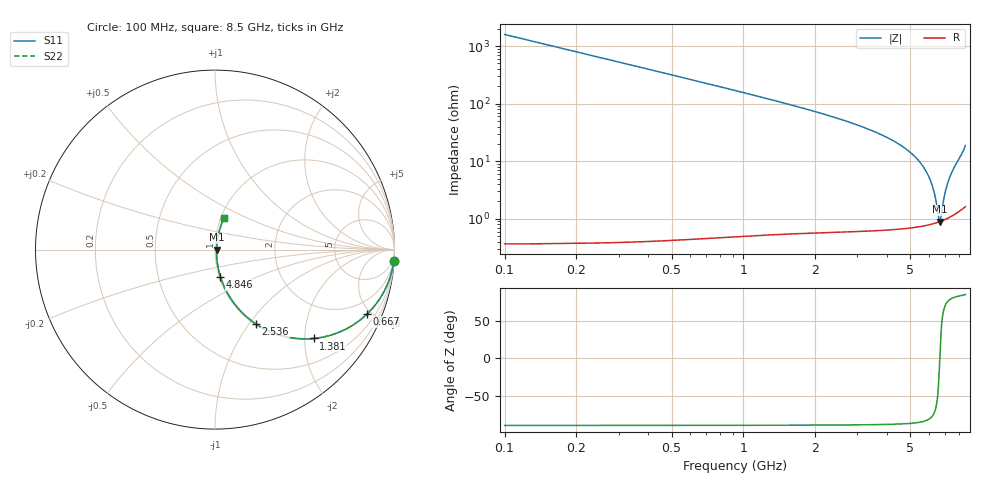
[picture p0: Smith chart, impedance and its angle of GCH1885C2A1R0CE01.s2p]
!Murata Part Number: GCH1885C2A1R0CE01
!These Parameters are Measured in Series Mode Connection
!Data Generated on Jun 19, 2026
!  o--ll--o
!Port1  Port2
!  o------o
!Operation Temp=25[degC], DC Bias Voltage=0[V]
!Freq. Start=100[MHz] Stop=9[GHz] 401[Steps]
# Hz S RI R 50
!Freq.(Hz) S11(Real) S11(Imag) S21(Real) S21(Imag) S12(Real) S12(Imag) S22(Real) S22(Imag)
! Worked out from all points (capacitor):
!   401 points, 100 MHz to 8.5 GHz, reference 50 ohm
!   read as one part in series: C = 1 pF near 142 MHz
!   lowest |Z| = 892 mohm at 6.631 GHz (marker M1)
!   series resonance near 6.64 GHz, so ESL is about 570 pH
!   S11 on the Smith chart (normalised r, x): 100 MHz: 1, -32; 667 MHz: 1.01, -4.72; 1.381 GHz: 1.01, -2.21; 2.536 GHz: 1.01, -1.08; 4.846 GHz: 1.01, -0.31; 8.5 GHz: 1.03, +0.37
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1e8  0.9961 -0.0626  0.00395 0.0626  0.00395 0.0626  0.9961 -0.0626
2.26e8  0.9801 -0.1393  0.0199 0.1393  0.0199 0.1393  0.9801 -0.1393
3.31e8  0.9582 -0.1998  0.0418 0.1998  0.0418 0.1998  0.9582 -0.1998
6.67e8  0.8475 -0.3585  0.1525 0.3585  0.1525 0.3585  0.8475 -0.3585
9.82e8  0.7148 -0.45  0.2852 0.45  0.2852 0.45  0.7148 -0.45
1.381e9  0.5489 -0.4952  0.4511 0.4952  0.4511 0.4952  0.5489 -0.4952
1.507e9  0.5014 -0.4973  0.4986 0.4973  0.4986 0.4973  0.5014 -0.4973
2.536e9  0.2274 -0.4137  0.7726 0.4137  0.7726 0.4137  0.2274 -0.4137
2.914e9  0.168 -0.3672  0.832 0.3672  0.832 0.3672  0.168 -0.3672
4.3e9  0.0513 -0.2063  0.9487 0.2063  0.9487 0.2063  0.0513 -0.2063
4.846e9  0.0305 -0.1516  0.9695 0.1516  0.9695 0.1516  0.0305 -0.1516
5.707e9  0.0131 -0.0744  0.9869 0.0744  0.9869 0.0744  0.0131 -0.0744
5.98e9  0.0105 -0.0518  0.9895 0.0518  0.9895 0.0518  0.0105 -0.0518
6.211e9  0.00922 -0.0333  0.9908 0.0333  0.9908 0.0333  0.00922 -0.0333
6.358e9  0.0088 -0.0217  0.9912 0.0217  0.9912 0.0217  0.0088 -0.0217
6.568e9  0.00872 -0.00553  0.9913 0.00553  0.9913 0.00553  0.00872 -0.00553
6.631e9  0.00881 -0.00072  0.9912 0.00072  0.9912 0.00072  0.00881 -0.00072
6.694e9  0.00896 0.00407  0.991 -0.00407  0.991 -0.00407  0.00896 0.00407
6.925e9  0.00992 0.0215  0.9901 -0.0215  0.9901 -0.0215  0.00992 0.0215
7.114e9  0.0112 0.0356  0.9888 -0.0356  0.9888 -0.0356  0.0112 0.0356
7.534e9  0.0159 0.0673  0.9841 -0.0673  0.9841 -0.0673  0.0159 0.0673
8.5e9  0.0481 0.1751  0.9519 -0.1751  0.9519 -0.1751  0.0481 0.1751
